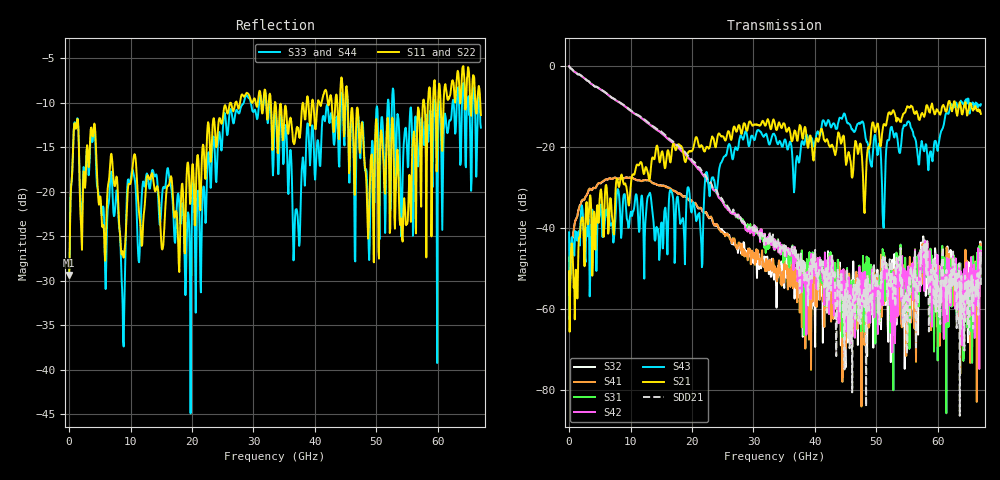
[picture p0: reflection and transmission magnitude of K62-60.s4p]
!Agilent Technologies,N5247A,US50470101,A.10.25.02
!Agilent N5247A: A.10.25.02
!Date: Tuesday, May 12, 2015 13:43:45
!Correction: Sdd11(Full 4 Port(1,2,3,4))
!Sdc11(Full 4 Port(1,2,3,4))
!Sdd12(Full 4 Port(1,2,3,4))
!Sdc12(Full 4 Port(1,2,3,4))
!Scd11(Full 4 Port(1,2,3,4))
!Scc11(Full 4 Port(1,2,3,4))
!Scd12(Full 4 Port(1,2,3,4))
!Scc12(Full 4 Port(1,2,3,4))
!Sdd21(Full 4 Port(1,2,3,4))
!Sdc21(Full 4 Port(1,2,3,4))
!Sdd22(Full 4 Port(1,2,3,4))
!Sdc22(Full 4 Port(1,2,3,4))
!Scd21(Full 4 Port(1,2,3,4))
!Scc21(Full 4 Port(1,2,3,4))
!Scd22(Full 4 Port(1,2,3,4))
!Scc22(Full 4 Port(1,2,3,4))
!Balanced Topology: BBAL
!S4P File: Measurements: <Sdd11,Sdc11,Sdd12,Sdc12>,
!<Scd11,Scc11,Scd12,Scc12>,
!<Sdd21,Sdc21,Sdd22,Sdc22>,
!<Scd21,Scc21,Scd22,Scc22>:
# Hz S  dB  R 50
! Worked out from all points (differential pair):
!   801 points, 10 MHz to 67 GHz, reference 50 ohm
!   strongest paths, dB at 10 MHz, 16.76 GHz, 33.51 GHz, 50.25 GHz, 67 GHz:
!     S21: -50.7, -20.6, -14.4, -14.2, -11.8
!     S43: -41.1, -31.2, -17.2, -21.7, -9.5
!     S42: -0.1, -18.8, -45.3, -66.2, -45.6
!     S31: -0.1, -18.8, -44.2, -53.2, -44.7
!     S41: -47.2, -30.6, -49.9, -59.5, -45.9
!     S32: -51.4, -30.6, -51.7, -54.6, -48.0
!   taken as a pair (ports 2,1 in; 4,3 out), SDD21 dB: 0.0, -18.5, -44.5, -60.9, -54.5
!   lowest |S11| = -29.4 dB at 10 MHz (marker M1), VSWR 1.07, Z = 50.2 + j3.4 ohm
!   |S11| at or under -10 dB: start of sweep to 27.06 GHz; 33.57 GHz to 38.65 GHz (5.081 GHz wide, 14.1 % of centre); 45.32 GHz to 57.59 GHz (12.26 GHz wide, 23.8 % of centre)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
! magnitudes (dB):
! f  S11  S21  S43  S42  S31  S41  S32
! 10 MHz  -29.4  -50.7  -41.1  -0.1  -0.1  -47.2  -51.4
! 9.975 GHz  -19.1  -30.6  -36.6  -11.0  -11.0  -27.5  -27.5
! 47.49 GHz  -13.4  -19.4  -14.0  -62.0  -65.5  -57.3  -57.7
! 51.17 GHz  -16.9  -14.4  -40.0  -50.3  -46.7  -55.3  -59.1
! 52.35 GHz  -18.3  -11.9  -15.2  -63.1  -55.6  -51.0  -73.1
! 64.49 GHz  -10.8  -8.9  -8.5  -62.2  -55.7  -45.3  -63.1
! 67 GHz  -11.4  -11.8  -9.5  -45.6  -44.7  -45.9  -48.0
